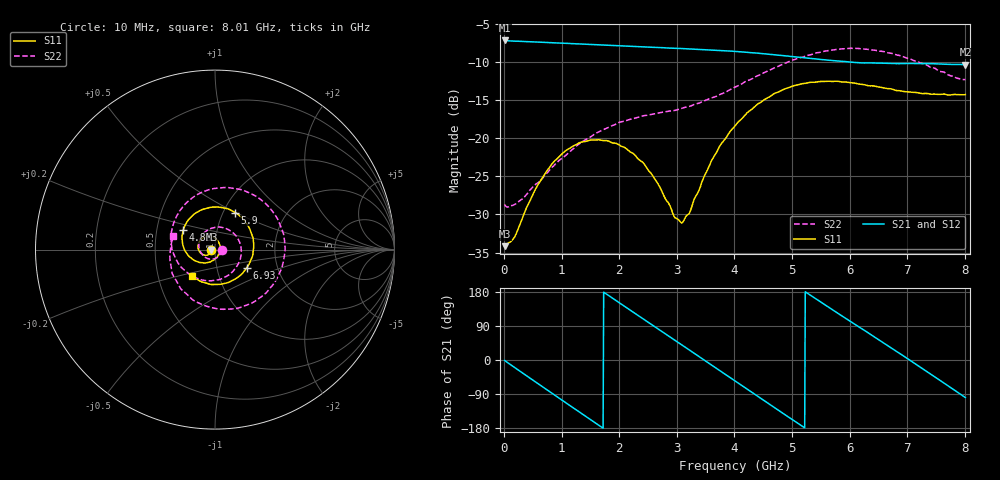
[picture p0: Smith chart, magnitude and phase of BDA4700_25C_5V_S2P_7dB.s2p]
!Agilent Technologies,E5071B,MY42404982,A.09.10
!Date: Mon Oct 20 13:29:28 2025
!Data & Calibration Information:
!Freq	S11:SOLT2(ON)	S21:SOLT2(ON)	S12:SOLT2(ON)	S22:SOLT2(ON)
# Hz S RI R 50
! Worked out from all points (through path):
!   801 points, 10 MHz to 8.01 GHz, reference 50 ohm
!   highest |S21| = -7.11 dB at 10 MHz (marker M1); lowest = -10.3 dB at 8.01 GHz (marker M2)
!   group delay of S21, straight-line fit = 283 ps
!   lowest |S11| = -34.2 dB at 10 MHz (marker M3), VSWR 1.04, Z = 48.1 - j0.0912 ohm
!   |S11| at or under -10 dB: start of sweep to end of sweep
!   |S22| runs from -29.0 to -8.1 dB; largest |S21 - S12| = 0.0034
!   S11 on the Smith chart (normalised r, x): 10 MHz: 0.96, -0.00; 4.83 GHz: 0.68, +0.16; 5.9 GHz: 1.14, +0.50; 6.93 GHz: 1.40, -0.29; 8.01 GHz: 0.74, -0.23
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1e7  -0.0196 -0.000948  0.4407 -0.00941  0.4409 -0.00989  0.0367 -0.00297
3.3e8  -0.0246 -0.0185  0.3548 -0.2502  0.3548 -0.2504  0.0231 -0.0331
7.2e8  -0.0501 -0.0315  0.103 -0.4154  0.103 -0.4154  -0.0231 -0.0531
1.02e9  -0.0771 -0.0219  -0.1258 -0.4037  -0.1263 -0.4042  -0.0672 -0.0326
1.35e9  -0.0944 0.00796  -0.327 -0.2592  -0.3276 -0.2592  -0.0902 0.0282
1.64e9  -0.0891 0.041  -0.4082 -0.0598  -0.4085 -0.0599  -0.0655 0.0887
1.93e9  -0.065 0.0665  -0.3788 0.1501  -0.3789 0.1504  -0.000172 0.1236
2.32e9  -0.0191 0.0714  -0.1901 0.3531  -0.1899 0.3534  0.1016 0.0929
2.68e9  0.0174 0.0465  0.0593 0.3916  0.0593 0.3914  0.1467 -0.00602
2.96e9  0.0284 0.0108  0.2372 0.3116  0.2374 0.311  0.1221 -0.0917
3.1e9  0.0266 -0.00864  0.3062 0.2411  0.3055 0.2422  0.0925 -0.1286
3.54e9  -0.0133 -0.0615  0.3799 -0.0455  0.3798 -0.0462  -0.0526 -0.1727
4.01e9  -0.101 -0.0664  0.2134 -0.307  0.2134 -0.3064  -0.2023 -0.0796
4.4e9  -0.1677 -0.00591  -0.0341 -0.3623  -0.0339 -0.3627  -0.245 0.0809
4.83e9  -0.1767 0.1101  -0.2671 -0.2282  -0.2662 -0.229  -0.1554 0.2641
5.35e9  -0.0686 0.2239  -0.3276 0.0707  -0.3279 0.07  0.1091 0.3403
5.9e9  0.1125 0.2063  -0.1247 0.2955  -0.1252 0.2951  0.3589 0.1487
6.28e9  0.1955 0.1104  0.0759 0.3044  0.0788 0.303  0.3774 -0.083
6.68e9  0.2111 -0.0254  0.2519 0.1831  0.2527 0.1827  0.2385 -0.2768
6.93e9  0.1774 -0.1005  0.3047 0.0607  0.3049 0.0592  0.0997 -0.3304
7.49e9  0.0248 -0.1938  0.2164 -0.2217  0.2157 -0.2221  -0.1946 -0.2122
8.01e9  -0.1281 -0.1461  -0.0487 -0.3017  -0.0484 -0.302  -0.2318 0.0745
